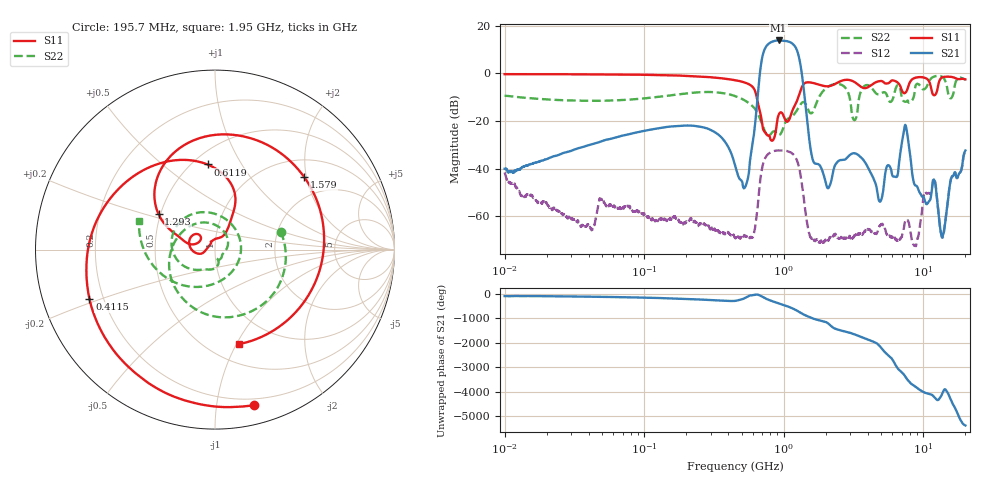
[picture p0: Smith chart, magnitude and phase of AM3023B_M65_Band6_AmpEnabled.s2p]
!Agilent Technologies,E8364B,MY43040894,A.07.50.67
!Agilent E8364B: A.07.50.67
!Date: Tuesday, October 27, 2020 10:53:39
!Correction: S11(Full 2 Port(1,2))
!S21(Full 2 Port(1,2))
!S12(Full 2 Port(1,2))
!S22(Full 2 Port(1,2))
!S2P File: Measurements: S11, S21, S12, S22:Log Frequency Sweep
# Hz S  dB  R 50
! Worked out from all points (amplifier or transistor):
!   3201 points, 10 MHz to 20 GHz, reference 50 ohm
!   highest |S21| = 13.9 dB at 918.5 MHz (marker M1)
!   |S21| within 3 dB of that: 739.3 MHz to 1.218 GHz (478.5 MHz wide, 48.9 % of centre)
!   unconditionally stable (mu >= 1): start of sweep to end of sweep
!   at 35.47 MHz: K = 2180.15, MAG = -19.9 dB, |S12| = -64.2 dB
!   at 447.2 MHz: K = 50630.00, MAG = -34.9 dB, |S12| = -69.0 dB
!   at 20 GHz: K = 177.80, MAG = -25.3 dB, |S12| = -32.8 dB
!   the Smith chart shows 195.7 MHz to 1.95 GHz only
!   S11 on the Smith chart (normalised r, x): 195.7 MHz: 0.15, -1.27; 411.5 MHz: 0.15, -0.19; 611.9 MHz: 0.59, +0.72; 1.293 GHz: 0.49, +0.22; 1.579 GHz: 1.41, +1.94; 1.95 GHz: 0.69, -1.03
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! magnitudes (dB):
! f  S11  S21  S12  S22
! 10 MHz  -0.3  -40.1  -41.6  -9.4
! 35.55 MHz  -0.4  -31.1  -63.8  -11.5
! 126.1 MHz  -0.7  -23.1  -61.5  -9.9
! 195.7 MHz  -1.0  -21.9  -62.9  -8.4
! 411.5 MHz  -2.5  -32.4  -67.6  -8.9
! 447.2 MHz  -2.8  -38.6  -69.0  -9.5
! 531.9 MHz  -3.9  -47.5  -68.4  -11.5
! 611.9 MHz  -6.4  -25.3  -66.9  -14.4
! 714.1 MHz  -23.7  8.7  -37.5  -22.6
! 918.5 MHz  -17.4  13.9  -32.4  -25.9
! 1.293 GHz  -8.6  6.1  -40.2  -13.8
! 1.579 GHz  -3.9  -33.9  -69.5  -16.8
! 1.59 GHz  -3.9  -34.8  -69.2  -16.6
! 1.95 GHz  -5.3  -43.5  -70.9  -6.9
! 3.289 GHz  -4.0  -33.7  -67.8  -18.8
! 4.902 GHz  -3.2  -53.9  -63.9  -8.6
! 5.639 GHz  -4.0  -38.6  -68.3  -11.2
! 7.481 GHz  -7.9  -22.0  -61.7  -11.9
! 8.772 GHz  -1.8  -47.1  -72.4  -5.4
! 11.92 GHz  -9.2  -44.7  -44.3  -1.3
! 13.68 GHz  -1.6  -68.9  -69.1  -1.5
! 20 GHz  -2.5  -32.4  -32.8  -2.6
